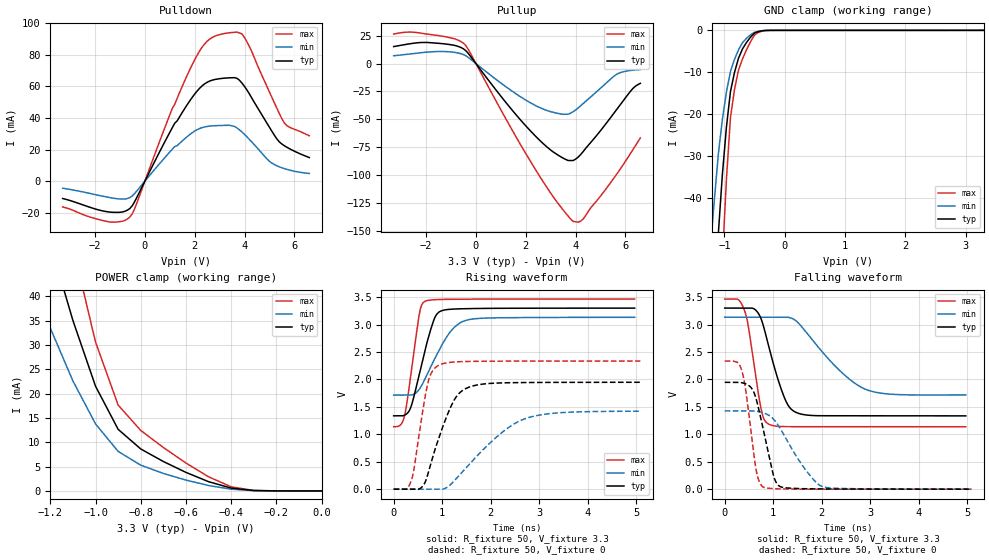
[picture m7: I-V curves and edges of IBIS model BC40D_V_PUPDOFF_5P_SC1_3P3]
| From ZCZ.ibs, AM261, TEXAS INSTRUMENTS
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[Model]   BC40D_V_PUPDOFF_5P_SC1_3P3
Model_type   I/O
Polarity   Non-Inverting
Enable   Active-Low
Vinl =  0.8V
Vinh =  2V
Cref =  15pF
Rref =  100.0000M
Vref =  0V
Vmeas =  1.65
C_comp   2.059994p   1.862014p   2.067327p
|[Input load] weak_pupdoff
|[Output drive] slow
|[supplytol] 5
|[temp] ind
[Model Spec]
Vinl   0.8V   0.8V   0.8V
Vinh   2V   2V   2V
[Temperature Range]   25   125   -40
[Voltage Range]   3.3   3.135   3.465
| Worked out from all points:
|   slope of the pulldown table from 0 to 0.495 V, typ, clamps not added: 31.8 ohm
|   slope of the pullup table from 0 to 0.495 V, typ, clamps not added: 33.8 ohm
|   GND clamp passes 1 mA (typ) near -0.53 V on its own axis
|   POWER clamp passes 1 mA (typ) near -0.43 V on its own axis
|   rising waveform, R_fixture 50, V_fixture 3.3: 20-80 % time 334ps typ, 511ps min, 217ps max; typ from 1.34 V to 3.3 V
|   rising waveform, R_fixture 50, V_fixture 0: 20-80 % time 466ps typ, 1.01ns min, 252ps max; typ from 0 V to 1.95 V
|   falling waveform, R_fixture 50, V_fixture 3.3: 20-80 % time 385ps typ, 889ps min, 239ps max; typ from 3.3 V to 1.34 V
|   falling waveform, R_fixture 50, V_fixture 0: 20-80 % time 293ps typ, 607ps min, 204ps max; typ from 1.95 V to 0 V
| Nom Voltages:
|   VDD=1.1, VDDS=3.3, VDDS18=1.8, ESD_BIASFET=0, VSS=0, VSSS=0
| Min Voltages:
|   VDD=1.045, VDDS=3.135, VDDS18=1.71, ESD_BIASFET=0, VSS=0, VSSS=0
| Max Voltages:
|   VDD=1.16, VDDS=3.465, VDDS18=1.89, ESD_BIASFET=0, VSS=0, VSSS=0
[POWER_clamp]
|   voltage   I(typ)   I(min)   I(max)
-3.3V     446.9mA    437.1mA    604mA
-1.267V   62.17mA    41.49mA    88.04mA
-1.233V   56.52mA    37.49mA    80.24mA
-1.133V   40.34mA    26.26mA    57.63mA
-1.067V   30.56mA    19.69mA    43.69mA
-1.033V   26.05mA    16.74mA    37.16mA
-1V       21.55mA    13.79mA    30.63mA
-900mV    12.68mA    8.13mA     17.66mA
-800mV    8.63mA     5.305mA    12.44mA
-600mV    3.813mA    2.231mA    5.735mA
-400mV    580.7uA    357.4uA    841.8uA
0V        4.589uA    2.331uA    8.159uA
[Pulldown]
|   voltage   I(typ)   I(min)   I(max)
-3.3V     -10.93mA   -4.474mA   -16.27mA
-1.4V     -19.53mA   -10.38mA   -25.83mA
-600mV    -17.23mA   -10.34mA   -22.61mA
1.2V      36.72mA    21.93mA    48.77mA
1.9V      53.02mA    30.66mA    73.76mA
2.4V      61.62mA    34.34mA    86.89mA
3V        64.86mA    35.24mA    92.76mA
3.6V      65.51mA    34.65mA    94.24mA
3.9V      62.01mA    31.1mA     93.16mA
5V        34.1mA     12.57mA    56.41mA
5.6V      22.42mA    7.958mA    36.79mA
6.6V      14.97mA    4.886mA    28.74mA
[Pullup]
|   voltage   I(typ)   I(min)   I(max)
-3.3V     15.12mA    6.907mA    26.36mA
-1.9V     18.73mA    10.27mA    26.12mA
-900mV    16.4mA     10.09mA    22.38mA
-400mV    11.39mA    6.888mA    15.9mA
1.3V      -37.44mA   -22.28mA   -53.31mA
2.4V      -65.08mA   -37.64mA   -95.03mA
3.3V      -81.9mA    -44.62mA   -125mA
3.9V      -86.71mA   -43.1mA    -141mA
4.3V      -78.82mA   -35.86mA   -139.1mA
5.6V      -42.54mA   -10.35mA   -100.4mA
6.3V      -22.29mA   -5.95mA    -77mA
6.6V      -17.71mA   -5.359mA   -66.44mA
[GND_clamp]
|   voltage   I(typ)   I(min)   I(max)
-3.3V     -787.2mA   -627.7mA   -1.235A
-1.233V   -85.66mA   -52.14mA   -138.8mA
-1.167V   -66.47mA   -40.37mA   -107.7mA
-1.1V     -48.25mA   -29.37mA   -77.98mA
-1.033V   -34.27mA   -21.19mA   -54.56mA
-966.7mV  -23.06mA   -14.66mA   -35.5mA
-900mV    -14.61mA   -9.789mA   -20.83mA
-833.3mV  -10.05mA   -6.934mA   -14.15mA
-700mV    -4.416mA   -2.931mA   -6.81mA
-500mV    -621.6uA   -443.6uA   -1.094mA
-300mV    -17.13uA   -24.35uA   -23.51uA
3.3V      4.589uA    5.188uA    6.318uA
[Ramp]
| variable   typ   min   max
dV/dt_f  1.1805738/0.38563216n 0.85640964/0.89611487n  1.3985723/0.23982487n
dV/dt_r  1.1742367/0.46733695n 0.86227327/1.0179189n  1.4069723/0.25275808n
R_load = 50
[Rising Waveform]
R_fixture = 50
V_fixture = 3.3
V_fixture_min = 3.135
V_fixture_max = 3.465
|   time   V(typ)   V(min)   V(max)
0s        1.337V     1.714V     1.139V
145.7ps   1.337V     1.714V     1.176V
223.8ps   1.348V     1.714V     1.335V
357.9ps   1.502V     1.715V     2.102V
531ps     2.107V     1.824V     3.197V
639.5ps   2.506V     1.995V     3.42V
907.4ps   3.206V     2.483V     3.456V
1.198ns   3.281V     2.899V     3.461V
1.485ns   3.29V      3.074V     3.463V
4.974ns   3.3V       3.132V     3.465V
[Rising Waveform]
R_fixture = 50
V_fixture = 0
V_fixture_min = 0
V_fixture_max = 0
|   time   V(typ)   V(min)   V(max)
0s        0V         0V         0V
262.4ps   0V         0V         0V
360.3ps   0V         0V         146mV
577.6ps   34.02mV    0V         1.301V
707.7ps   278.1mV    0V         1.94V
932ps     934.7mV    0V         2.258V
1.271ns   1.657V     173.1mV    2.32V
1.624ns   1.879V     514.9mV    2.33V
2.781ns   1.944V     1.304V     2.335V
5.091ns   1.948V     1.421V     2.335V
[Falling Waveform]
R_fixture = 50
V_fixture = 3.3
V_fixture_min = 3.135
V_fixture_max = 3.465
|   time   V(typ)   V(min)   V(max)
0s        3.3V       3.134V     3.464V
276.8ps   3.3V       3.134V     3.457V
412.9ps   3.3V       3.134V     3.247V
752.2ps   3.102V     3.134V     1.455V
907.9ps   2.605V     3.134V     1.184V
1.248ns   1.634V     3.134V     1.14V
1.512ns   1.385V     3.036V     1.138V
2.313ns   1.338V     2.213V     1.138V
2.894ns   1.337V     1.824V     1.138V
4.974ns   1.336V     1.717V     1.138V
[Falling Waveform]
R_fixture = 50
V_fixture = 0
V_fixture_min = 0
V_fixture_max = 0
|   time   V(typ)   V(min)   V(max)
0s        1.947V     1.427V     2.334V
357.1ps   1.939V     1.427V     2.148V
438.8ps   1.917V     1.427V     1.773V
649.9ps   1.641V     1.423V     344mV
797ps     1.084V     1.391V     37.23mV
1.02ns    214.2mV    1.264V     8.723mV
1.175ns   37mV       1.06V      4.37mV
1.658ns   7.631mV    364.9mV    0V
2.028ns   4.359mV    43.7mV     0V
5.091ns   0V         2.16mV     0V
